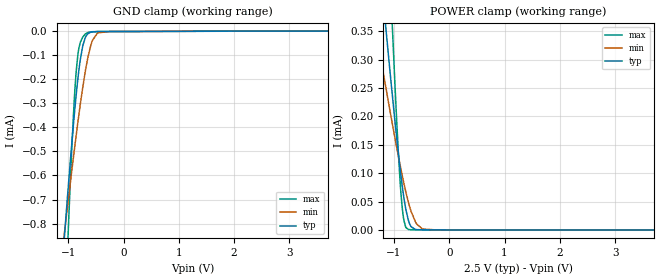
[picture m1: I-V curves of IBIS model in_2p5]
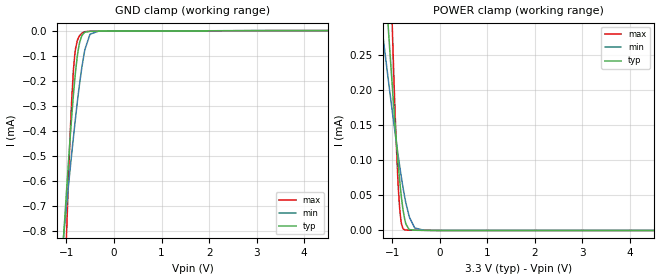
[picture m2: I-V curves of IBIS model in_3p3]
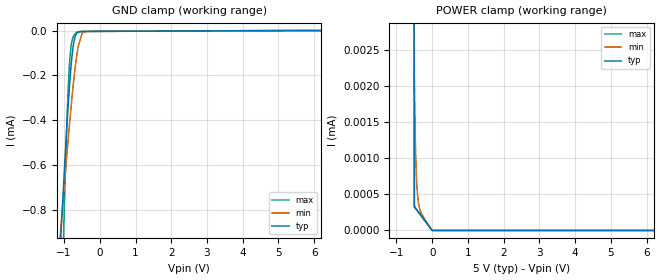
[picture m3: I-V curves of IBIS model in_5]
|Texas Instruments Incorporated
| High-Performance, 5.7kVRMS Reinforced Quad Channel Digital Isolators.
| Marketing part#   Digital Voltage Range   Package-type   #pins
| IS07742DW   2.25V-5.5V   SOIC   16
| IS07742DWR   2.25V-5.5V   SOIC   16
| IS07742DBQ   2.25V-5.5V   SOIC   16
| IS07742DBQR   2.25V-5.5V   SOIC   16
| IS07742FDW   2.25V-5.5V   SOIC   16
| IS07742FDWR   2.25V-5.5V   SOIC   16
| IS07742FDBQ   2.25V-5.5V   SOIC   16
| IS07742FDBQR   2.25V-5.5V   SOIC   16
[IBIS Ver]   4.1
[File name]   iso7742.ibs
[File Rev]   1.1
[Date]   9/19/2017
[Source]
| Texas Instruments Incorporated.
| Analog-eLab Design Center, HPA
| 12500 TI Blvd
| Dallas, TX -75243
[Notes]   Revision History:
| Rev 1.0: 5/10/2016
| - Initial version of the model
| Rev 1.1: 9/19/2017
| - Add DBQ package component
| - Model based on ISO7841
| - C_comp although listed in numerical order of value are
|   obtained from varying PVT conditions. For PVT conditions for
|   each specific value refer the buffer description under
|   respective [Model]. IBIS model user is responsible for using
|   appropriate C_comp to simulate for Signal Integrity.
|* EXCEPTION:   *
|* - For in_* and en_* models there will be leakage current in   *
|*   GROUND clamp because of a resistor(RH2) connected to pad.   *
|* - For inf_* models there will be leakage current in POWER clamp  *
|*   because of a resistor(R1) connected to pad.   *
[Disclaimer]
| This model is designed as an aid for customers of Texas Instruments.
| TI and its licensors and suppliers make no warranties, either expressed
| or implied, with respect to this  model, including the warranties of
| merchantability or fitness for a particular purpose. The model is
| provided solely on an "as is" basis. The entire risk as to its quality
| and performance is with the customer.
[Copyright]
(C) Copyright 2017 Texas Instruments Incorporated.All rights reserved.
|   IS07742DW
[Component]   IS07742DW
[Manufacturer]   TI
[Package]   |16 SOIC - DW package
|   typ   min   max
R_pkg   0.13983   0.12494   0.17928
L_pkg   2.1802nH   1.92454nH   2.85707nH
C_pkg   0.42060pF   0.21450pF   0.61276pF
[Pin]  signal_name   model_name   R_pin   L_pin   C_pin
1   VCC1   POWER   0.09703   2.25823nH  0.63889pF
2   GND1   GND   0.10567   2.15194nH  0.30706pF
3   INA   IN   0.12889   1.99554nH  0.21450pF
4   INB   IN   0.12623   1.94755nH  0.61276pF
5   INC   IN   0.12494   1.92646nH  0.36666pF
6   OUTD   OUT   0.14038   2.18765nH  0.43235pF
7   EN1   EN   0.17807   2.83638nH  0.45904pF
8   GND1   GND   0.08216   2.43955nH  0.44498pF
9   GND2   GND   0.10126   2.44074nH  0.40934pF
10   EN2   EN   0.17928   2.85707nH  0.52717pF
11   IND   IN   0.12883   1.99615nH  0.50841pF
12   OUTC   OUT   0.12617   1.94399nH  0.32633pF
13   OUTB   OUT   0.12498   1.92454nH  0.37783pF
14   OUTA   OUT   0.14050   2.18615nH  0.38097pF
15   GND2   GND   0.08275   2.09014nH  0.75096pF
16   VCC2   POWER   0.09747   2.26909nH  0.67439pF
|   IS07742FDW
[Component]   IS07742FDW
[Manufacturer]   TI
[Package]   |16 SOIC - DW package
|   typ   min   max
R_pkg   0.13983   0.12494   0.17928
L_pkg   2.1802nH   1.92454nH   2.85707nH
C_pkg   0.42060pF   0.21450pF   0.61276pF
[Pin]  signal_name   model_name   R_pin   L_pin   C_pin
1   VCC1   POWER   0.09703   2.25823nH  0.63889pF
2   GND1   GND   0.10567   2.15194nH  0.30706pF
3   INA   INF   0.12889   1.99554nH  0.21450pF
4   INB   INF   0.12623   1.94755nH  0.61276pF
5   INC   INF   0.12494   1.92646nH  0.36666pF
6   OUTD   OUT   0.14038   2.18765nH  0.43235pF
7   EN1   EN   0.17807   2.83638nH  0.45904pF
8   GND1   GND   0.08216   2.43955nH  0.44498pF
9   GND2   GND   0.10126   2.44074nH  0.40934pF
10   EN2   EN   0.17928   2.85707nH  0.52717pF
11   IND   INF   0.12883   1.99615nH  0.50841pF
12   OUTC   OUT   0.12617   1.94399nH  0.32633pF
13   OUTB   OUT   0.12498   1.92454nH  0.37783pF
14   OUTA   OUT   0.14050   2.18615nH  0.38097pF
15   GND2   GND   0.08275   2.09014nH  0.75096pF
16   VCC2   POWER   0.09747   2.26909nH  0.67439pF
|   IS07742DBQ
[Component]   IS07742DBQ
[Manufacturer]   TI
[Package]   |16 SOIC - DBQ package
|   typ   min   max
R_pkg   0.102   0.056   0.131
L_pkg   1.26E-09H   6.63E-10H   1.48E-09H
C_pkg   3.11E-13F   1.29E-13F   2.19E-12F
[Pin]  signal_name   model_name   R_pin   L_pin   C_pin
1   VCC1   POWER   0.0794   9.954E-10H   2.185E-12F
2   GND1   GND   0.0635   1.126E-09H   2.016E-13F
3   INA   IN   0.1143   1.378E-09H   1.321E-13F
4   INB   IN   0.1132   1.342E-09H   1.399E-13F
5   OUTC   OUT   0.1128   1.294E-09H   1.403E-13F
6   OUTD   OUT   0.1181   1.337E-09H   1.404E-13F
7   EN1   EN   0.1311   1.465E-09H   1.404E-13F
8   GND1   GND   0.0883   1.313E-09H   2.153E-13F
9   GND2   GND   0.0988   1.354E-09H   2.174E-13F
10   EN2   EN   0.1302   1.483E-09H   1.402E-13F
11   IND   IN   0.1162   1.387E-09H   1.396E-13F
12   INC   IN   0.1132   1.350E-09H   1.287E-13F
13   OUTB   OUT   0.1119   1.304E-09H   2.578E-13F
14   OUTA   OUT   0.1155   1.331E-09H   2.020E-13F
15   GND2   GND   0.0673   1.078E-09H   2.034E-13F
16   VCC2   POWER   0.0563   6.633E-10H   3.885E-13F
|   IS07742FDBQ
[Component]   IS07742FDBQ
[Manufacturer]   TI
[Package]   |16 SOIC - DBQ package
|   typ   min   max
R_pkg   0.102   0.056   0.131
L_pkg   1.26E-09H   6.63E-10H   1.48E-09H
C_pkg   3.11E-13F   1.29E-13F   2.19E-12F
[Pin]  signal_name   model_name   R_pin   L_pin   C_pin
1   VCC1   POWER   0.0794   9.954E-10H   2.185E-12F
2   GND1   GND   0.0635   1.126E-09H   2.016E-13F
3   INA   INF   0.1143   1.378E-09H   1.321E-13F
4   INB   INF   0.1132   1.342E-09H   1.399E-13F
5   OUTC   OUT   0.1128   1.294E-09H   1.403E-13F
6   OUTD   OUT   0.1181   1.337E-09H   1.404E-13F
7   EN1   EN   0.1311   1.465E-09H   1.404E-13F
8   GND1   GND   0.0883   1.313E-09H   2.153E-13F
9   GND2   GND   0.0988   1.354E-09H   2.174E-13F
10   EN2   EN   0.1302   1.483E-09H   1.402E-13F
11   IND   INF   0.1162   1.387E-09H   1.396E-13F
12   INC   INF   0.1132   1.350E-09H   1.287E-13F
13   OUTB   OUT   0.1119   1.304E-09H   2.578E-13F
14   OUTA   OUT   0.1155   1.331E-09H   2.020E-13F
15   GND2   GND   0.0673   1.078E-09H   2.034E-13F
16   VCC2   POWER   0.0563   6.633E-10H   3.885E-13F
|   Model Selectors
[Model Selector] EN
en_2p5   2.5V digital Input
en_3p3   3.3V digital Input
en_5   5.0V digital Input
[Model Selector] IN
in_2p5   2.5V digital Input
in_3p3   3.3V digital Input
in_5   5.0V digital Input
[Model Selector] INF
inf_2p5   2.5V digital Input
inf_3p3   3.3V digital Input
inf_5   5.0V digital Input
[Model Selector] OUT
out_2p5   2.5V digital 3-state
out_3p3   3.3V digital 3-state
out_5   5.0V digital 3-state
| Models and submodels in the file (12): in_2p5 (Input), in_3p3 (Input), in_5 (Input), inf_2p5 (Input), inf_3p3 (Input), inf_5 (Input), en_2p5 (Input), en_3p3 (Input), en_5 (Input), out_2p5 (3-state), out_3p3 (3-state), out_5 (3-state)
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|   in_2p5 Model
[Model]   in_2p5
Model_type   Input
Vinl = 0.75
Vinh = 1.75
|   typ   min   max
|   (nom PVT)   (fast PVT)   (slow PVT)
C_comp   3.281e-15   3.281e-15   3.250e-14
[Model spec]
|subparameter
Vinl   0.75   0.675   0.825
Vinh   1.75   1.575   1.925
| Where nom  PVT is Nominal Process, 2.5V, 27C
|   Fast PVT is Strong Process,  2.75V, -55C
|   Slow PVT is Weak Process,   2.25V, 150C
[Voltage Range]   2.5   2.25   2.75
|Ambient Temperature   25   125   -55
|Junction Temperature
[Temperature Range]   27   150   -55
[Power Clamp Reference]   2.5   2.25   2.75
[GND Clamp Reference]   0   0   0
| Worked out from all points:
|   GND clamp passes 1 mA (typ) near -1.12 V on its own axis
[GND Clamp]
|   Voltage   I(typ)   I(min)   I(max)
-2.5V     -5.567mA   -3.855mA   -11.2mA
-1.071V   -859.9uA   -843.3uA   -1.249mA
-1.015V   -691.9uA   -732.5uA   -914.2uA
-965mV    -547.7uA   -635.6uA   -635.6uA
-894mV    -356.2uA   -501.7uA   -297uA
-827.5mV  -201.6uA   -381.9uA   -101.5uA
-737.5mV  -61.36uA   -233.7uA   -24.74uA
-643.8mV  -10.62uA   -108.8uA   -5.86uA
-564mV    -3.337uA   -39.15uA   -2.62uA
-468.2mV  -2.078uA   -7.417uA   -2.095uA
-250mV    -1.826uA   -1.892uA   -1.932uA
5V        0A         0A         0A
[POWER Clamp]
|   Voltage   I(typ)   I(min)   I(max)
-2.5V     1.812mA    1.039mA    3.985mA
-1.351V   565.2uA    364.2uA    1.113mA
-1.196V   404.1uA    277.3uA    740.6uA
-1.053V   258.8uA    198.6uA    407.1uA
-990.2mV  197.6uA    165uA      269.2uA
-924.3mV  136.7uA    131uA      139.5uA
-874.8mV  94.88uA    106.6uA    63.72uA
-822.5mV  56.84uA    82.23uA    17.11uA
-740mV    16.82uA    48.51uA    910.2nA
-612.5mV  771.4nA    14.03uA    395.2nA
-486.3mV  326.4nA    1.63uA     313.2nA
5V        0A         0A         0A
|   in_3p3 Model
[Model]   in_3p3
Model_type   Input
Vinl = 0.99
Vinh = 2.31
|   typ   min   max
|   (nom PVT)   (fast PVT)   (slow PVT)
C_comp   3.281e-15   3.281e-15   3.329e-14
[Model spec]
|subparameter
Vinl   0.99   0.891   1.089
Vinh   2.31   2.079   2.541
| Where nom  PVT is Nominal Process, 3.3V, 27C
|   Fast PVT is Strong Process,  3.63V, -55C
|   Slow PVT is Weak Process,   2.97V, 150C
[Voltage Range]   3.3   2.97   3.63
|Ambient Temperature   25   125   -55
|Junction Temperature
[Temperature Range]   27   150   -55
[Power Clamp Reference]   3.3   2.97   3.63
[GND Clamp Reference]   0   0   0
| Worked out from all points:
|   GND clamp passes 1 mA (typ) near -1.12 V on its own axis
|   POWER clamp passes 1 mA (typ) near -1.76 V on its own axis
[GND Clamp]
|   Voltage   I(typ)   I(min)   I(max)
-3.3V     -8.284mA   -5.57mA    -16.97mA
-1.076V   -873.8uA   -852.4uA   -1.277mA
-1.002V   -654.6uA   -707.6uA   -841.1uA
-893.3mV  -354.6uA   -500.5uA   -294.5uA
-853.4mV  -258.1uA   -427.8uA   -159.9uA
-825mV    -196.7uA   -377.6uA   -97.46uA
-772.2mV  -104.4uA   -288.5uA   -41.12uA
-722.7mV  -47.98uA   -211.7uA   -20.38uA
-620.4mV  -7.55uA    -84.56uA   -4.818uA
-505.2mV  -2.819uA   -14.66uA   -2.744uA
-330mV    -2.413uA   -2.673uA   -2.551uA
6.6V      0A         0A         0A
[POWER Clamp]
|   Voltage   I(typ)   I(min)   I(max)
-3.3V     2.693mA    1.517mA    6.009mA
-1.242V   451.1uA    302.7uA    849uA
-1.198V   405.5uA    278.1uA    743.9uA
-1.049V   255uA      196.5uA    398.4uA
-965.9mV  174.7uA    152.3uA    218.9uA
-878.8mV  98.13uA    108.5uA    68.84uA
-842.5mV  70.44uA    91.34uA    30.66uA
-805.2mV  46.22uA    74.6uA     9.403uA
-737.2mV  15.94uA    47.51uA    852.4nA
-526mV    364.9nA    3.505uA    338.9nA
-330mV    219.3nA    268.9nA    212.6nA
6.6V      0A         0A         0A
|   in_5 Model
[Model]   in_5
Model_type   Input
Vinl = 1.5
Vinh = 3.5
|   typ   min   max
|   (nom PVT)   (fast PVT)   (slow PVT)
C_comp   3.281e-15   3.281e-15   3.455e-14
[Model spec]
|subparameter
Vinl   1.5   1.35   1.65
Vinh   3.5   3.15   3.85
| Where nom  PVT is Nominal Process, 5V, 27C
|   Fast PVT is Strong Process,  5.5V, -55C
|   Slow PVT is Weak Process,   4.5V, 150C
[Voltage Range]   5   4.5   5.5
|Ambient Temperature   25   125   -55
|Junction Temperature
[Temperature Range]   27   150   -55
[Power Clamp Reference]   5   4.5   5.5
[GND Clamp Reference]   0   0   0
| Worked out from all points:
|   GND clamp passes 1 mA (typ) near -1.12 V on its own axis
[GND Clamp]
|   Voltage   I(typ)   I(min)   I(max)
-5V       -13.99mA   -9.044mA   -29.25mA
-1.112V   -984.6uA   -924.8uA   -1.503mA
-1.062V   -832.2uA   -825.1uA   -1.194mA
-974mV    -573.5uA   -653.1uA   -684.8uA
-908mV    -392.7uA   -527.9uA   -356.7uA
-850mV    -250.8uA   -421.9uA   -151.8uA
-809mV    -166.1uA   -350.2uA   -74.38uA
-740mV    -65.1uA    -237.9uA   -26.95uA
-608mV    -7.374uA   -73.42uA   -5.426uA
-500mV    -3.903uA   -14.37uA   -3.931uA
-338mV    -3.55uA    -3.864uA   -3.762uA
10V       0A         0A         0A
[POWER Clamp]
|   Voltage   I(typ)   I(min)   I(max)
-5V       185.5mA    66.86mA    305.6mA
-1.007V   213.6uA    173.9uA    305uA
-500mV    338.3nA    2.124uA    322.2nA
-482mV    323.5nA    1.505uA    310.6nA
-473mV    316.7nA    1.273uA    304.8nA
-459.5mV  306.8nA    1.002uA    296.1nA
-432.5mV  288nA      655.7nA    278.7nA
-396.5mV  263.7nA    427.3nA    255.5nA
-360.5mV  239.7nA    320.4nA    232.3nA
-306.5mV  203.8nA    241.2nA    197.5nA
-500uV    0A         0A         0A
10V       0A         0A         0A
